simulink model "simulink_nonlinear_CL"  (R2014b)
settings: Solver=ode45  StartTime=0.0  StopTime=10.0  RelTol=1e-3

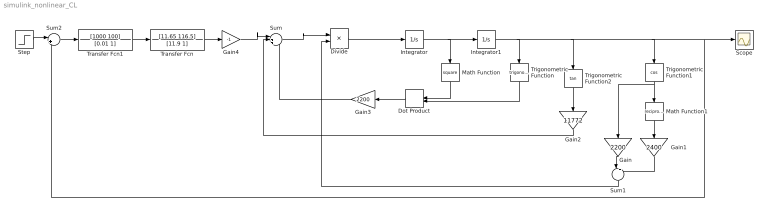
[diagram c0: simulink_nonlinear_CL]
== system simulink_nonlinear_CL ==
  Divide : Product  Inputs=*/
  Dot Product : DotProduct
  Gain : Gain  Gain=2200
  Gain1 : Gain  Gain=2400
  Gain2 : Gain  Gain=11772
  Gain3 : Gain  Gain=2200
  Gain4 : Gain  Gain=-1
  Integrator : Integrator
  Integrator1 : Integrator
  Math Function : Math  Operator=square
  Math Function1 : Math  Operator=reciprocal
  Scope : Scope
  Step : Step  Time=0  SampleTime=0
  Sum : Sum  Inputs=|+++
  Sum1 : Sum  Inputs=|+-
  Sum2 : Sum  Inputs=|+-
  Transfer Fcn : TransferFcn  Numerator=[11.65 116.5]  Denominator=[11.9 1]
  Transfer Fcn1 : TransferFcn  Numerator=[1000 100]  Denominator=[0.01 1]
  Trigonometric Function : Trigonometry
  Trigonometric Function1 : Trigonometry  Operator=cos
  Trigonometric Function2 : Trigonometry  Operator=tan
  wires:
  Sum/1 -> Divide/1
  Divide/1 -> Integrator/1
  Integrator/1 -> Math Function/1, Integrator1/1
  Integrator1/1 -> Sum2/2, Scope/1, Trigonometric Function1/1, Trigonometric Function2/1, Trigonometric Function/1
  Math Function/1 -> Dot Product/1
  Trigonometric Function/1 -> Dot Product/2
  Dot Product/1 -> Gain3/1
  Trigonometric Function1/1 -> Gain/1, Math Function1/1
  Math Function1/1 -> Gain1/1
  Gain/1 -> Sum1/1
  Gain1/1 -> Sum1/2
  Sum1/1 -> Divide/2
  Trigonometric Function2/1 -> Gain2/1
  Gain2/1 -> Sum/2
  Gain3/1 -> Sum/3
  Step/1 -> Sum2/1
  Transfer Fcn/1 -> Gain4/1
  Sum2/1 -> Transfer Fcn1/1
  Transfer Fcn1/1 -> Transfer Fcn/1
  Gain4/1 -> Sum/1
